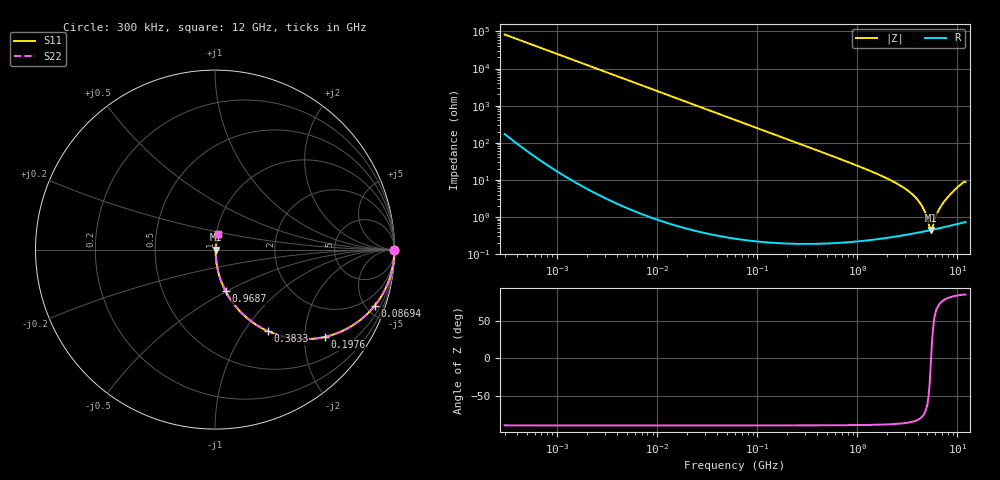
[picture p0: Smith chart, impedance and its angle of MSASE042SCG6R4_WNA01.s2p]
! MSASE042SCG6R4_WNA01  S-PARAMETER MODEL  ( General Type )
! Model Generated by TAIYO YUDEN Corporation (http://www.ty-top.com)
! Version 1.0
! TAIYO YUDEN Control No. 130801
! Copyright(c) 2013 TAIYO YUDEN CO.,LTD. All Rights Reserved.
! Product Description (link to TY-COMPAS)
! https://ds.yuden.co.jp/TYCOMPAS/or/detail?pn=MSASE042SCG6R4BWNA01&u=M
! Products Name : Multilayer Ceramic Capacitors
! Characteristics :
!  Capacitance : 6.4 pF , Rated Voltage : 16V , TCC : CG / C0G
!  Case Size : 0.4 x 0.2 / 0.016 x 0.008 [mm/inch] , Thickness : 0.2 / 0.008 [mm/inch]
!  (Conditions: Temperature = 25 degC , DC Bias Current/Voltage = 0A / 0V)
! External Node Assignments :
!  1  o---| |---o  2
! GND o---------o GND
! Frequency Range : 0.3MHz  -  12000MHz  [ 401 STEP ]
# MHz S RI R 50
! Freq[MHz].  S11 Real  S11 Imag  S21 Real  S21 Imag  S12 Real  S12 Imag  S22 Real  S22 Imag
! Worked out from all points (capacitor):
!   401 points, 300 kHz to 12 GHz, reference 50 ohm
!   read as one part in series: C = 6.41 pF near 316.3 kHz
!   lowest |Z| = 444 mohm at 5.42 GHz (marker M1)
!   series resonance near 5.452 GHz, so ESL is about 130 pH
!   S11 on the Smith chart (normalised r, x): 300 kHz: open; 86.94 MHz: 1.00, -5.71; 197.6 MHz: 1.00, -2.51; 383.3 MHz: 1.00, -1.29; 968.7 MHz: 1.00, -0.50; 12 GHz: 1.01, +0.17
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0.3  1 -0.00121  3.96e-06 0.00121  3.96e-06 0.00121  1 -0.00121
1.769972  0.9999 -0.00713  5.43e-05 0.00713  5.43e-05 0.00713  0.9999 -0.00713
10.44266  0.9982 -0.042  0.00178 0.042  0.00178 0.042  0.9982 -0.042
27.10171  0.9882 -0.1079  0.0118 0.1079  0.0118 0.1079  0.9882 -0.1079
60  0.9446 -0.2284  0.0554 0.2284  0.0554 0.2284  0.9446 -0.2284
86.94074  0.8904 -0.312  0.1096 0.312  0.1096 0.312  0.8904 -0.312
197.6437  0.6111 -0.4867  0.3889 0.4867  0.3889 0.4867  0.6111 -0.4867
353.9943  0.3281 -0.4682  0.6719 0.4682  0.6719 0.4682  0.3281 -0.4682
383.2761  0.2939 -0.4541  0.7061 0.4541  0.7061 0.4541  0.2939 -0.4541
601.3112  0.1437 -0.3484  0.8563 0.3484  0.8563 0.3484  0.1437 -0.3484
968.706  0.0598 -0.2327  0.9402 0.2327  0.9402 0.2327  0.0598 -0.2327
2088.533  0.0129 -0.0998  0.9871 0.0998  0.9871 0.0998  0.0129 -0.0998
3026.31  0.00643 -0.0562  0.9936 0.0562  0.9936 0.0562  0.00643 -0.0562
3944.255  0.00459 -0.0297  0.9954 0.0297  0.9954 0.0297  0.00459 -0.0297
4502.883  0.00427 -0.0174  0.9957 0.0174  0.9957 0.0174  0.00427 -0.0174
5140.631  0.00429 -0.0053  0.9957 0.0053  0.9957 0.0053  0.00429 -0.0053
5420.343  0.00439 -0.000475  0.9956 0.000475  0.9956 0.000475  0.00439 -0.000475
5715.274  0.00454 0.00391  0.9955 -0.00391  0.9955 -0.00391  0.00454 0.00391
6524.734  0.0051 0.0146  0.9949 -0.0146  0.9949 -0.0146  0.0051 0.0146
7648.807  0.00621 0.0287  0.9938 -0.0287  0.9938 -0.0287  0.00621 0.0287
10236.47  0.0107 0.0648  0.9893 -0.0648  0.9893 -0.0648  0.0107 0.0648
12000  0.0145 0.085  0.9855 -0.085  0.9855 -0.085  0.0145 0.085
